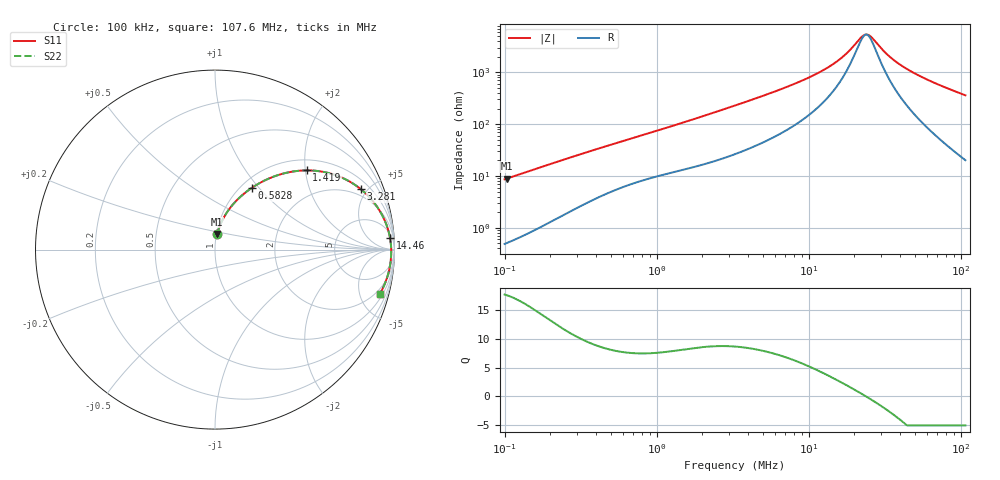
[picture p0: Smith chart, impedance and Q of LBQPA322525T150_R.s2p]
! LBQPA322525T150_R  S-PARAMETER MODEL  ( General Type )
! Model Generated by TAIYO YUDEN Corporation (http://www.ty-top.com)
! Version 1.0
! TAIYO YUDEN Control No. 191025NI43SB-FBB
! Copyright(c) 2019 TAIYO YUDEN CO.,LTD. All Rights Reserved.
! Product Description (link to TY-COMPAS)
! https://ds.yuden.co.jp/TYCOMPAS/or/detail?pn=LBQPA322525T150KR&u=M
! Products Name : Inductors
! Characteristics :
!  Inductance : 15 uH , SRF(min) : 20 MHz , DC Resistance(max) : 0.2535 Ohm
!  Rated Current : Saturation :730 mA , Temp Rise : 590 mA (20 degC)
!  Case Size : 3.2 x 2.5 / 0.126 x 0.098 [mm/inch] , Thickness : 2.5 / 0.098 [mm/inch]
!  (Conditions: Temperature = 25 degC , DC Bias Current/Voltage = 0A / 0V)
! External Node Assignments :
!  1  o---GGG---o  2
! GND o---------o GND
! Frequency Range : 0.1MHz  -  107.617193MHz  [ 402 STEP ]
# MHz S RI R 50
! Freq[MHz].  S11 Real  S11 Imag  S21 Real  S21 Imag  S12 Real  S12 Imag  S22 Real  S22 Imag
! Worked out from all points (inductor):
!   401 points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, 100 kHz to 107.6 MHz, reference 50 ohm
!   read as one part in series: L = 13.7 uH near 103.6 kHz
!   highest Q = 17.5 at 103.6 kHz (marker M1), where L = 13.7 uH
!   self-resonance near 23.93 MHz
!   S11 on the Smith chart (normalised r, x): 100 kHz: 1.01, +0.17; 582.8 kHz: 1.12, +0.91; 1.419 MHz: 1.25, +2.04; 3.281 MHz: 1.53, +4.56; 14.46 MHz: 10, +27; 107.6 MHz: 1.40, -7.21
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0.1  0.0122 0.0848  0.9878 -0.0848  0.9878 -0.0848  0.0122 0.0848
0.103552  0.0129 0.0877  0.9871 -0.0877  0.9871 -0.0877  0.0129 0.0877
0.194101  0.0379 0.157  0.9621 -0.157  0.9621 -0.157  0.0379 0.157
0.321988  0.088 0.2372  0.912 -0.2372  0.912 -0.2372  0.088 0.2372
0.582841  0.204 0.3433  0.796 -0.3433  0.796 -0.3433  0.204 0.3433
1.036765  0.3863 0.4253  0.6137 -0.4253  0.6137 -0.4253  0.3863 0.4253
1.419433  0.5113 0.4413  0.4887 -0.4413  0.4887 -0.4413  0.5113 0.4413
2.08386  0.6667 0.4166  0.3333 -0.4166  0.3333 -0.4166  0.6667 0.4166
3.280506  0.8138 0.3356  0.1862 -0.3356  0.1862 -0.3356  0.8138 0.3356
6.257342  0.9276 0.199  0.0724 -0.199  0.0724 -0.199  0.9276 0.199
10.56285  0.9652 0.1083  0.0348 -0.1083  0.0348 -0.1083  0.9652 0.1083
14.46158  0.9755 0.0636  0.0245 -0.0636  0.0245 -0.0636  0.9755 0.0636
17.83085  0.9793 0.0364  0.0207 -0.0364  0.0207 -0.0364  0.9793 0.0364
22.37218  0.9815 0.00827  0.0185 -0.00827  0.0185 -0.00827  0.9815 0.00827
23.98983  0.9818 -0.000303  0.0182 0.000303  0.0182 0.000303  0.9818 -0.000303
24.842  0.9819 -0.00459  0.0181 0.00459  0.0181 0.00459  0.9819 -0.00459
26.17735  0.9819 -0.0111  0.0181 0.0111  0.0181 0.0111  0.9819 -0.0111
34.01114  0.9807 -0.0443  0.0193 0.0443  0.0193 0.0443  0.9807 -0.0443
41.20956  0.9781 -0.0704  0.0219 0.0704  0.0219 0.0704  0.9781 -0.0704
53.54187  0.9713 -0.11  0.0287 0.11  0.0287 0.11  0.9713 -0.11
74.59468  0.9542 -0.1695  0.0458 0.1695  0.0458 0.1695  0.9542 -0.1695
107.6172  0.9167 -0.2497  0.0833 0.2497  0.0833 0.2497  0.9167 -0.2497
